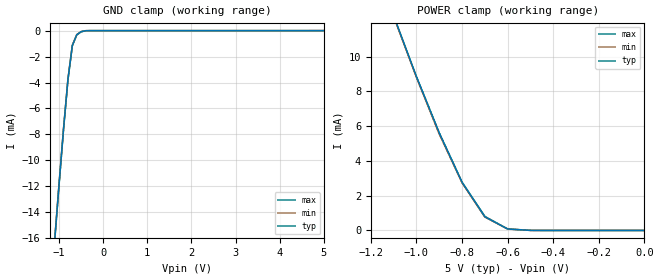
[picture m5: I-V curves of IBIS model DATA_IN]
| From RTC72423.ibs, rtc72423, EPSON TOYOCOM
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[Model]   DATA_IN
Model_type   Input
Polarity   Non-Inverting
Vinl =   0.8V
Vinh =   2.2V
C_comp   0.80pF   0.60pF   1.00pF
[Temperature Range]   25.00   85.00   -40.00
[Voltage Range]   5.0V   4.5V   5.50V
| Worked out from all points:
|   GND clamp passes 1 mA (typ) near -0.68 V on its own axis
|   POWER clamp passes 1 mA (typ) near -0.71 V on its own axis
[GND_clamp]
| voltage   I(typ)   I(min)   I(max)
-5V       -171.2mA   -169.8mA   -170.9mA
-1.1V     -16.19mA   -16.13mA   -16.22mA
-1V       -11.82mA   -11.76mA   -11.86mA
-900mV    -7.606mA   -7.564mA   -7.653mA
-800mV    -3.782mA   -3.743mA   -3.821mA
-700mV    -1.149mA   -1.122mA   -1.169mA
-600mV    -313uA     -306uA     -333uA
-500mV    -78uA      -74uA      -90uA
-300mV    0A         0A         0A
5V        0A         5uA        0A
[POWER_clamp]
| voltage   I(typ)   I(min)   I(max)
-5V       163.9mA    164.8mA    164.2mA
-1.1V     12.34mA    12.29mA    12.33mA
-1V       8.837mA    8.791mA    8.84mA
-900mV    5.599mA    5.538mA    5.612mA
-800mV    2.766mA    2.739mA    2.785mA
-700mV    786uA      772uA      810uA
-600mV    86uA       83uA       88uA
-500mV    5uA        5uA        5uA
0V        0A         0A         0A
